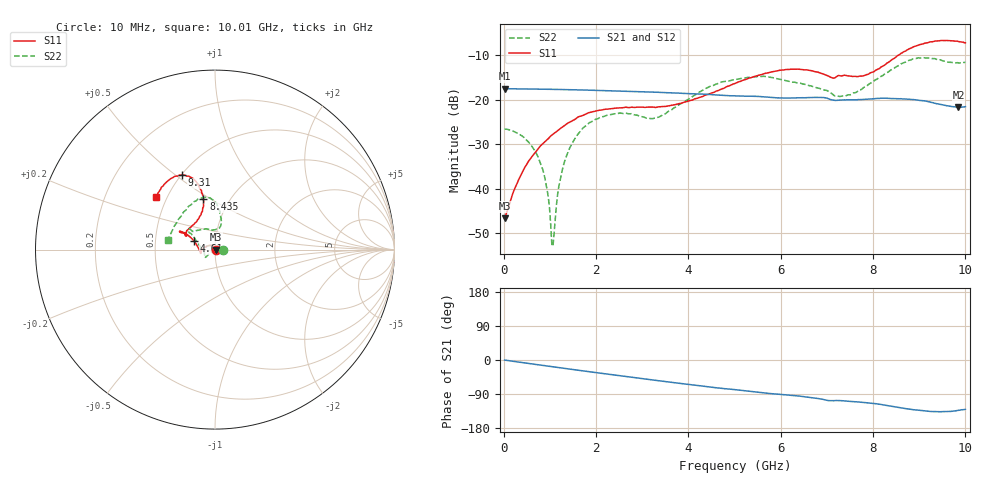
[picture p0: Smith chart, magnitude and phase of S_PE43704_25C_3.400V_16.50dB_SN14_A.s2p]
! Device ID: PE43704
! Dir: z:\PE43704\PE43704_Char_1_20130516\PE43704\AMB\3p400V\16p50dB
! Serial: 14
! Insertion: A
! Impedance: 50 ohm
! Temp: Amb
! VDD: 3.400V
! Attenuation Step: 16.50dB
! IDD: 1.139219e-01mA
#  Hz  S  RI  R  50
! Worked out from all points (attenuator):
!   401 points, 10 MHz to 10.01 GHz, reference 50 ohm
!   highest |S21| = -17.47 dB at 10 MHz (marker M1); lowest = -21.6 dB at 9.86 GHz (marker M2)
!   lowest |S11| = -46.6 dB at 10 MHz (marker M3), VSWR 1.01, Z = 50.5 + j0.0392 ohm
!   |S11| at or under -10 dB: start of sweep to 8.545 GHz
!   |S22| runs from -52.9 to -10.5 dB; largest |S21 - S12| = 0.0012
!   S11 on the Smith chart (normalised r, x): 10 MHz: 1.01, +0.00; 4.61 GHz: 0.79, +0.08; 8.435 GHz: 0.76, +0.46; 9.31 GHz: 0.51, +0.53; 10.01 GHz: 0.44, +0.32
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1e7  0.00465 0.000388  0.1338 -0.000428  0.1339 -0.00048  0.0471 -2.5e-06
3.6e8  2.36e-05 0.0142  0.1325 -0.0145  0.1323 -0.0147  0.0399 0.00508
7.1e8  -0.0141 0.023  0.1295 -0.0277  0.1294 -0.0277  0.0238 0.00554
8.85e8  -0.0239 0.024  0.1274 -0.0342  0.1274 -0.0341  0.0128 0.00287
1.01e9  -0.0313 0.0238  0.1259 -0.0387  0.1259 -0.0386  0.00399 -0.00017
1.06e9  -0.0343 0.0228  0.1252 -0.0405  0.1253 -0.0404  0.000475 -0.00223
1.185e9  -0.0413 0.0207  0.1232 -0.045  0.1233 -0.0449  -0.00821 -0.00661
1.285e9  -0.0469 0.0185  0.1216 -0.0484  0.1216 -0.0483  -0.0152 -0.0103
1.685e9  -0.0661 0.00532  0.114 -0.0613  0.1141 -0.0613  -0.0375 -0.0278
2.36e9  -0.0785 -0.0156  0.0983 -0.08  0.0983 -0.0798  -0.0545 -0.0429
3.36e9  -0.0829 -0.0125  0.0701 -0.0995  0.0702 -0.0994  -0.0638 -0.0075
4.61e9  -0.1171 0.0473  0.0326 -0.109  0.0329 -0.1089  -0.1273 0.0814
5.01e9  -0.137 0.0686  0.0225 -0.1088  0.0227 -0.1088  -0.1417 0.0927
5.96e9  -0.1888 0.1011  -0.000626 -0.1056  -0.000341 -0.1055  -0.1332 0.108
6.685e9  -0.1901 0.095  -0.0173 -0.1052  -0.0174 -0.1049  -0.0922 0.1081
7.385e9  -0.1582 0.1048  -0.0311 -0.0953  -0.0307 -0.0952  -0.00319 0.1104
7.835e9  -0.0991 0.1631  -0.039 -0.094  -0.0389 -0.0939  0.0321 0.1376
8.36e9  -0.0635 0.2616  -0.0539 -0.0891  -0.054 -0.0896  0.0281 0.2087
8.435e9  -0.0643 0.2812  -0.056 -0.0873  -0.056 -0.0876  0.0215 0.2213
9.31e9  -0.1834 0.4138  -0.0674 -0.0642  -0.0673 -0.0641  -0.1088 0.2705
9.86e9  -0.302 0.337  -0.0564 -0.0608  -0.0569 -0.06  -0.2349 0.1131
1.001e10  -0.3278 0.2915  -0.0542 -0.0643  -0.0551 -0.064  -0.2605 0.0509
